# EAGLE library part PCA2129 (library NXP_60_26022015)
Accurate RTC with integrated quartz crystal for industrial The PCF2129T is a CMOS1 Real Time Clock (RTC) and calendar with an integrated Temperature Compensated Crystal (Xtal) Oscillator (TCXO) and a 32.768 kHz quartz crystal optimized for very high accuracy and very low power consumption. The PCF2129T has a selectable I2C-bus or SPI-bus, a backup battery switch-over circuit, a programmable watchdog function, a timestamp function, and many other features. AAL Eindhoven MK
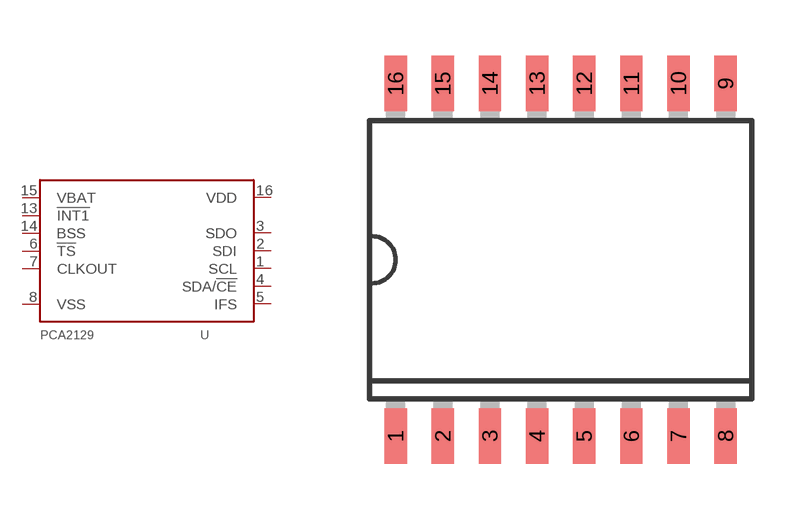
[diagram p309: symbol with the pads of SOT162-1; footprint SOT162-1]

Designator prefix U

## PCA2129T (TEMPERATURE_RANGE: -30 °C to +80 °C)  [SOT162-1]
1  SCL
2  SDI  in
3  SDO  out
4  SDA/!CE  in
5  IFS  in
6  !TS!  in
7  CLKOUT  out
8  VSS  pwr
13  !INT1!  out
14  BSS  out
15  VBAT  pwr
16  VDD  pwr

## Footprint SOT162-1 (pad centres in mm)
SOT162-1 SO16: plastic small outline package; 16 leads; body width 7.5 mm JEDEC: -- IEC: --
smd 0.6 x 1.5: 1 -4.445,-4.75; 2 -3.175,-4.75; 3 -1.905,-4.75; 4 -0.635,-4.75; 5 0.635,-4.75; 6 1.905,-4.75; 7 3.175,-4.75; 8 4.445,-4.75; 9 4.445,4.75; 10 3.175,4.75; 11 1.905,4.75; 12 0.635,4.75; 13 -0.635,4.75; 14 -1.905,4.75; 15 -3.175,4.75; 16 -4.445,4.75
